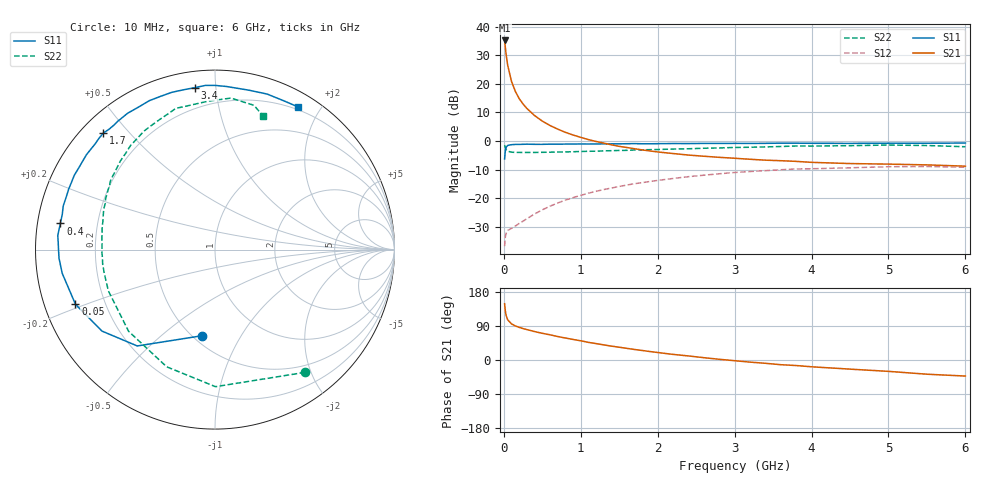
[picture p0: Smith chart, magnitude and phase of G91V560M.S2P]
! SIEMENS Small Signal Semiconductors
! BFG235
! Si NPN RF Bipolar Junction Transistor in SOT223
! VCE = 1.5 V  IC = 60 mA
! Common Emitter S-Parameters:  July  1994
# GHz  S  MA  R  50
!  f  S11  S21  S12  S22
! GHz  MAG  ANG  MAG  ANG  MAG  ANG  MAG  ANG
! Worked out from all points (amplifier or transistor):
!   40 points, 10 MHz to 6 GHz, reference 50 ohm
!   highest |S21| = 35.1 dB at 10 MHz (marker M1)
!   |S21| within 3 dB of that: start of sweep to 21.83 MHz
!   unconditionally stable (mu >= 1): 464.4 MHz to 1.598 GHz
!   at 200 MHz: K = 0.71, MSG = 21.8 dB, |S12| = -28.8 dB
!   at 1.5 GHz: K = 1.02, MAG = 6.1 dB, |S12| = -15.9 dB
!   at 6 GHz: K = 0.94, MSG = 0.2 dB, |S12| = -9.2 dB
!   S11 on the Smith chart (normalised r, x): 10 MHz: 0.55, -0.69; 50 MHz: 0.09, -0.19; 400 MHz: 0.07, +0.08; 1.7 GHz: 0.06, +0.43; 3.4 GHz: 0.08, +0.88; 6 GHz: 0.17, +1.73
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0.01  0.4859 -98.8  57.13 148.5  0.0145 60.1  0.8485 -53.7
0.02  0.6898 -128.9  42.51 128.9  0.0214 42.9  0.7637 -89.8
0.03  0.7763 -144.2  32.37 117.4  0.0244 35.0  0.7064 -112.4
0.05  0.835 -158.6  21.03 106.1  0.0273 28.1  0.6624 -136.6
0.1  0.8615 -171.2  10.95 95.3  0.0297 28.5  0.637 -158.8
0.15  0.8703 -176.8  7.336 89.8  0.0326 34.4  0.6309 -167.7
0.2  0.8718 -179.9  5.49 86.1  0.0362 38.7  0.6311 -172.5
0.25  0.8747 177.2  4.42 82.9  0.0397 43.2  0.6288 -176.0
0.3  0.8795 174.9  3.695 80.3  0.0438 46.3  0.6304 -178.8
0.4  0.8737 170.4  2.78 75.0  0.053 50.4  0.6301 177.3
0.5  0.8733 167.0  2.225 70.5  0.0626 53.1  0.6335 174.1
0.6  0.8799 164.0  1.862 66.5  0.0724 54.3  0.6365 171.2
0.7  0.8791 160.4  1.612 61.9  0.0824 55.0  0.6413 168.6
0.9  0.8831 154.9  1.272 54.2  0.1023 53.9  0.6486 163.9
1.1  0.8852 148.5  1.056 46.5  0.1222 51.9  0.6606 159.3
1.7  0.8991 133.8  0.731 27.7  0.1793 42.9  0.6958 147.1
2.2  0.9023 122.6  0.603 14.8  0.221 34.0  0.7225 136.8
3.2  0.9075 101.2  0.479 -5.6  0.2923 14.8  0.7766 117.4
3.4  0.9092 97.1  0.462 -8.7  0.303 10.9  0.7871 113.2
4.5  0.908 78.1  0.403 -24.1  0.3397 -9.5  0.8275 92.8
5.5  0.9134 65.2  0.382 -37.5  0.3576 -27.2  0.8328 74.9
6  0.9199 59.7  0.363 -42.4  0.3468 -33.8  0.7922 70.3
